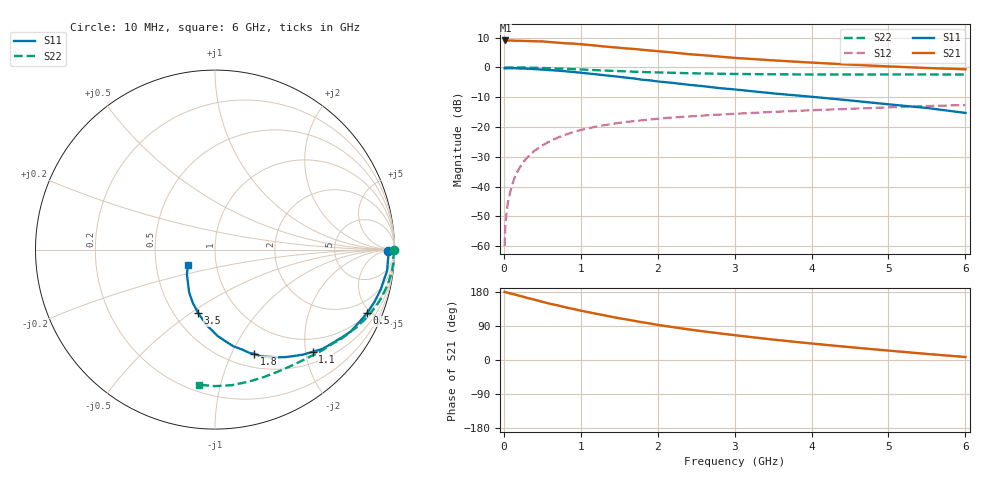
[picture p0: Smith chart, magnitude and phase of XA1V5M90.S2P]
! SIEMENS Discrete & RF Semiconductors
! BFY180
! Si NPN RF Bipolar Junction Transistor in MICRO-X
! VCE = 1.5 V  IC = 0.9 mA
! Common Emitter S-Parameters:  May  1997
# GHz  S  MA  R  50
!  f  S11  S21  S12  S22
! GHz  MAG  ANG  MAG  ANG  MAG  ANG  MAG  ANG
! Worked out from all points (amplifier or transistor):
!   36 points, 10 MHz to 6 GHz, reference 50 ohm
!   highest |S21| = 9.0 dB at 20 MHz (marker M1)
!   |S21| within 3 dB of that: start of sweep to 1.753 GHz
!   unconditionally stable (mu >= 1): 3.629 GHz to end of sweep
!   at 250 MHz: K = 0.08, MSG = 20.4 dB, |S12| = -31.9 dB
!   at 1.4 GHz: K = 0.52, MSG = 12.9 dB, |S12| = -19.0 dB
!   at 6 GHz: K = 1.08, MAG = 4.3 dB, |S12| = -12.6 dB
!   S11 on the Smith chart (normalised r, x): 10 MHz: 52, -10; 500 MHz: 1.06, -4.76; 1.1 GHz: 0.71, -2.14; 1.8 GHz: 0.65, -1.22; 3.5 GHz: 0.66, -0.54; 6 GHz: 0.73, -0.13
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0.01  0.9635 -0.4  2.802 179.7  0.001 87.5  0.9986 -0.2
0.02  0.9599 -0.9  2.827 178.9  0.0024 95.9  0.9993 -0.6
0.05  0.9665 -2.0  2.803 177.6  0.0052 81.3  0.9973 -1.3
0.1  0.9653 -4.8  2.825 174.9  0.0101 89.1  0.9942 -2.7
0.15  0.9663 -7.0  2.788 172.4  0.0153 85.6  0.9976 -4.1
0.3  0.9502 -13.5  2.768 164.1  0.0303 79.8  0.9895 -8.1
0.5  0.9178 -22.7  2.723 153.6  0.0488 74.0  0.9756 -13.2
0.6  0.8995 -26.7  2.658 148.4  0.0579 71.0  0.9663 -15.7
0.9  0.8358 -38.7  2.506 134.8  0.0818 62.4  0.9336 -22.7
1.1  0.7877 -46.3  2.378 126.2  0.0948 57.8  0.9087 -26.9
1.2  0.7643 -49.9  2.316 122.0  0.1014 55.0  0.8982 -29.0
1.5  0.694 -59.9  2.134 110.2  0.1172 49.1  0.865 -34.5
1.8  0.6202 -69.4  1.972 99.5  0.1295 44.6  0.8355 -39.4
2  0.5802 -74.4  1.87 92.6  0.1373 41.5  0.8224 -42.6
2.2  0.5479 -79.3  1.772 86.7  0.1444 38.7  0.8106 -45.6
2.4  0.5107 -83.9  1.667 80.8  0.1496 36.5  0.7972 -48.4
2.8  0.4487 -92.3  1.517 70.4  0.1612 32.5  0.7808 -53.8
3.5  0.3659 -104.8  1.31 53.9  0.179 26.3  0.7648 -62.8
4  0.3212 -112.7  1.202 43.5  0.1909 22.1  0.7605 -69.3
4.5  0.2788 -121.1  1.112 33.9  0.2018 18.3  0.7591 -75.9
5.5  0.2083 -138.7  0.976 16.0  0.2239 10.2  0.7607 -89.9
6  0.172 -150.9  0.928 7.9  0.2332 6.1  0.7578 -96.9
